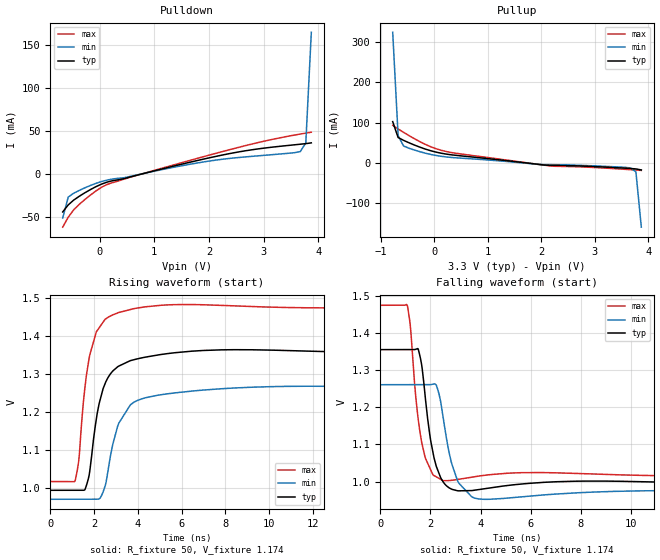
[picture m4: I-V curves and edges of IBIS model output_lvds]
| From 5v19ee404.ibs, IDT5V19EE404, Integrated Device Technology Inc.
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|   Model output_lvds
[Model]   output_lvds
Model_type   Output
Polarity   Non-Inverting
|   typ   min   max
C_comp   2pF   1.5pF   2.5pF
Vmeas = 1.13V
Rref = 50
Cref = 0
Vref = 1.13V
|   typ   min   max
[Voltage range]   3.3V   3.135V   3.465V
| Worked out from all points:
|   slope of the pulldown table from 0 to 0.495 V, typ, clamps not added: 59.8 ohm
|   slope of the pullup table from 0 to 0.495 V, typ, clamps not added: 47.6 ohm
|   rising waveform, R_fixture 50, V_fixture 1.174: 20-80 % time 714ps typ, 929ps min, 613ps max; typ from 0.993 V to 1.35 V
|   falling waveform, R_fixture 50, V_fixture 1.174: 20-80 % time 432ps typ, 501ps min, 405ps max; typ from 1.35 V to 0.993 V
[Pulldown]
|Voltage   I (typ)   I (min)   I (max)
|Note, modeling breaks down at 250mA and above.  This is well beyond the functional   |
|operating range of the device.  Should this scenario occur, catastrophic failure and   |
|possible damage to the device and/or board is of higher concern than the I-V curve   |
|behavior.  The IBIS checker will flag currents in excess of 10A with warnings.  Lines   |
|with currents in excess of 0.35 A have been commented out.  The points still remain|
|available to the user if the user desires to use them.   |
|-3.30000e+00   -6.87685e+01   -5.43171e+01   -9.32007e+01
|-3.19898e+00   -6.58202e+01   -5.20452e+01   -8.91014e+01
|-3.09796e+00   -6.28734e+01   -4.97746e+01   -8.50038e+01
|-2.99694e+00   -5.99283e+01   -4.75054e+01   -8.09081e+01
|-2.89592e+00   -5.69849e+01   -4.52379e+01   -7.68145e+01
|-2.79490e+00   -5.40436e+01   -4.29720e+01   -7.27232e+01
|-2.69388e+00   -5.11045e+01   -4.07081e+01   -6.86346e+01
|-2.59286e+00   -4.81679e+01   -3.84464e+01   -6.45488e+01
|-2.49184e+00   -4.52340e+01   -3.61870e+01   -6.04662e+01
|-2.39082e+00   -4.23033e+01   -3.39304e+01   -5.63874e+01
|-2.28980e+00   -3.93762e+01   -3.16768e+01   -5.23129e+01
|-2.18878e+00   -3.64533e+01   -2.94267e+01   -4.82434e+01
|-2.08776e+00   -3.35351e+01   -2.71806e+01   -4.41796e+01
|-1.98673e+00   -3.06226e+01   -2.49393e+01   -4.01228e+01
|-1.88571e+00   -2.77168e+01   -2.27034e+01   -3.60743e+01
|-1.78469e+00   -2.48193e+01   -2.04743e+01   -3.20362e+01
|-1.68367e+00   -2.19318e+01   -1.82533e+01   -2.80115e+01
|-1.58265e+00   -1.90572e+01   -1.60423e+01   -2.40041e+01
|-1.48163e+00   -1.61996e+01   -1.38443e+01   -2.00194e+01
|-1.38061e+00   -1.33650e+01   -1.16633e+01   -1.60669e+01
|-1.27959e+00   -1.05641e+01   -9.50588e+00   -1.21633e+01
|-1.17857e+00   -7.81468e+00   -7.38281e+00   -8.34234e+00
|-1.07755e+00   -5.15408e+00   -5.31429e+00   -4.68989e+00
|-9.76531e-01   -2.67976e+00   -3.34319e+00   -1.52157e+00
|-8.75510e-01   -7.34230e-01   -1.58050e+00   -1.40830e-01
|-7.74490e-01   -8.44745e-02   -3.68373e-01   -7.56037e-02
-673.5mV  -44.12mA   -51.13mA   -61.81mA
-572.4mV  -35.88mA   -26.81mA   -50.24mA
-471.4mV  -30.25mA   -22.24mA   -41.53mA
-370.4mV  -25.84mA   -19mA      -35.27mA
33.67mV   -11.77mA   -8.741mA   -15.46mA
538.8mV   -3.726mA   -3.071mA   -4.119mA
1.448V    10.68mA    9.012mA    12.28mA
2.256V    22.28mA    17.32mA    26.32mA
2.862V    28.96mA    21.02mA    36.12mA
3.67V     34.74mA    26.19mA    46.58mA
3.771V    35.43mA    36.18mA    47.67mA
3.872V    36.31mA    165mA      48.72mA
| 3.97347e+00   3.90604e-02   7.21592e-01   4.97824e-02
| 4.07449e+00   7.95512e-02   1.56794e+00   5.12016e-02
| 4.17551e+00   5.50354e-01   2.52334e+00   5.37009e-02
| 4.27653e+00   1.56933e+00   3.52849e+00   6.05171e-02
| 4.37755e+00   2.77655e+00   4.56116e+00   2.90811e-01
| 4.47857e+00   4.05579e+00   5.61110e+00   1.44560e+00
| 4.57959e+00   5.37132e+00   6.67281e+00   2.97907e+00
| 4.68061e+00   6.70844e+00   7.74304e+00   4.62016e+00
| 4.78163e+00   8.05979e+00   8.81972e+00   6.30839e+00
| 4.88265e+00   9.42118e+00   9.90143e+00   8.02268e+00
| 4.98367e+00   1.07900e+01   1.09873e+01   9.75343e+00
| 5.08469e+00   1.21646e+01   1.20769e+01   1.14955e+01
| 5.18571e+00   1.35438e+01   1.31697e+01   1.32457e+01
| 5.28673e+00   1.49267e+01   1.42651e+01   1.50023e+01
| 5.38776e+00   1.63127e+01   1.53626e+01   1.67637e+01
| 5.48878e+00   1.77013e+01   1.64619e+01   1.85291e+01
| 5.58980e+00   1.90921e+01   1.75627e+01   2.02978e+01
| 5.69082e+00   2.04848e+01   1.86650e+01   2.20692e+01
| 5.79184e+00   2.18792e+01   1.97684e+01   2.38429e+01
| 5.89286e+00   2.32754e+01   2.08729e+01   2.56187e+01
| 5.99388e+00   2.46734e+01   2.19784e+01   2.73961e+01
| 6.09490e+00   2.60729e+01   2.30848e+01   2.91751e+01
| 6.19592e+00   2.74736e+01   2.41920e+01   3.09553e+01
| 6.29694e+00   2.88754e+01   2.52999e+01   3.27368e+01
| 6.39796e+00   3.02780e+01   2.64085e+01   3.45193e+01
| 6.49898e+00   3.16814e+01   2.75177e+01   3.63028e+01
| 6.60000e+00   3.30855e+01   2.86274e+01   3.80871e+01
[Pullup]
|Voltage   I (typ)   I (min)   I (max)
|Note, modeling breaks down at 250mA and above.  This is well beyond the functional   |
|operating range of the device.  Should this scenario occur, catastrophic failure and   |
|possible damage to the device and/or board is of higher concern than the I-V curve   |
|behavior.  The IBIS checker will flag currents in excess of 10A with warnings.  Lines   |
|with currents in excess of 0.35 A have been commented out.  The points still remain|
|available to the user if the user desires to use them.   |
|-3.30000e+00   3.30649e+01   2.68016e+01   4.09786e+01
|-3.19898e+00   3.16617e+01   2.56933e+01   3.91941e+01
|-3.09796e+00   3.02592e+01   2.45857e+01   3.74103e+01
|-2.99694e+00   2.88577e+01   2.34787e+01   3.56274e+01
|-2.89592e+00   2.74574e+01   2.23726e+01   3.38453e+01
|-2.79490e+00   2.60586e+01   2.12672e+01   3.20642e+01
|-2.69388e+00   2.46610e+01   2.01628e+01   3.02842e+01
|-2.59286e+00   2.32645e+01   1.90595e+01   2.85054e+01
|-2.49184e+00   2.18693e+01   1.79573e+01   2.67280e+01
|-2.39082e+00   2.04756e+01   1.68564e+01   2.49522e+01
|-2.28980e+00   1.90836e+01   1.57571e+01   2.31782e+01
|-2.18878e+00   1.76934e+01   1.46596e+01   2.14063e+01
|-2.08776e+00   1.63054e+01   1.35644e+01   1.96368e+01
|-1.98673e+00   1.49200e+01   1.24719e+01   1.78702e+01
|-1.88571e+00   1.35377e+01   1.13822e+01   1.61071e+01
|-1.78469e+00   1.21590e+01   1.02955e+01   1.43482e+01
|-1.68367e+00   1.07850e+01   9.21254e+00   1.25947e+01
|-1.58265e+00   9.41664e+00   8.13421e+00   1.08481e+01
|-1.48163e+00   8.05582e+00   7.06175e+00   9.11072e+00
|-1.38061e+00   6.70508e+00   5.99695e+00   7.38625e+00
|-1.27959e+00   5.36863e+00   4.94257e+00   5.68119e+00
|-1.17857e+00   4.05393e+00   3.90315e+00   4.00831e+00
|-1.07755e+00   2.77593e+00   2.88682e+00   2.39814e+00
|-9.76531e-01   1.57108e+00   1.91017e+00   9.53385e-01
|-8.75510e-01   5.58820e-01   1.01408e+00   1.52918e-01
-774.5mV  102.2mA    323.4mA    93.03mA
-673.5mV  62.84mA    67.73mA    84.09mA
-572.4mV  55.86mA    41.9mA     75.76mA
-370.4mV  44.27mA    31.88mA    60.01mA
-67.35mV  30.17mA    20.96mA    40.14mA
134.7mV   23.86mA    16.26mA    31.05mA
336.7mV   19.73mA    13.3mA     25.29mA
2.155V    -6.05mA    -4.394mA   -7.483mA
2.963V    -8.992mA   -7.283mA   -11.27mA
3.67V     -13.9mA    -12.54mA   -16.81mA
3.771V    -15mA      -22.29mA   -17.68mA
3.872V    -17.52mA   -159.3mA   -18.74mA
| 3.97347e+00   -2.33400e-02   -1.03894e+00   -2.12284e-02
| 4.07449e+00   -6.44071e-02   -2.66328e+00   -2.74433e-02
| 4.17551e+00   -7.26444e-01   -4.57897e+00   -3.69091e-02
| 4.27653e+00   -2.67901e+00   -6.61921e+00   -5.08167e-02
| 4.37755e+00   -5.15548e+00   -8.72536e+00   -3.22188e-01
| 4.47857e+00   -7.81696e+00   -1.08716e+01   -2.57527e+00
| 4.57959e+00   -1.05668e+01   -1.30445e+01   -5.99938e+00
| 4.68061e+00   -1.33678e+01   -1.52365e+01   -9.73121e+00
| 4.78163e+00   -1.62020e+01   -1.74427e+01   -1.35885e+01
| 4.88265e+00   -1.90591e+01   -1.96600e+01   -1.75125e+01
| 4.98367e+00   -2.19330e+01   -2.18859e+01   -2.14777e+01
| 5.08469e+00   -2.48198e+01   -2.41190e+01   -2.54708e+01
| 5.18571e+00   -2.77167e+01   -2.63580e+01   -2.94842e+01
| 5.28673e+00   -3.06217e+01   -2.86020e+01   -3.35131e+01
| 5.38776e+00   -3.35335e+01   -3.08503e+01   -3.75539e+01
| 5.48878e+00   -3.64509e+01   -3.31022e+01   -4.16042e+01
| 5.58980e+00   -3.93731e+01   -3.53574e+01   -4.56623e+01
| 5.69082e+00   -4.22995e+01   -3.76153e+01   -4.97268e+01
| 5.79184e+00   -4.52294e+01   -3.98758e+01   -5.37968e+01
| 5.89286e+00   -4.81625e+01   -4.21385e+01   -5.78715e+01
| 5.99388e+00   -5.10984e+01   -4.44032e+01   -6.19502e+01
| 6.09490e+00   -5.40367e+01   -4.66697e+01   -6.60325e+01
| 6.19592e+00   -5.69773e+01   -4.89378e+01   -7.01179e+01
| 6.29694e+00   -5.99199e+01   -5.12074e+01   -7.42060e+01
| 6.39796e+00   -6.28643e+01   -5.34784e+01   -7.82967e+01
| 6.49898e+00   -6.58103e+01   -5.57507e+01   -8.23896e+01
| 6.60000e+00   -6.87579e+01   -5.80241e+01   -8.64845e+01
[Ramp]
|   typ   min   max
dV/dt_r   0.222/0.774n   0.178/0.949n   0.28/0.643n
dV/dt_f   0.229/0.48n   0.186/0.577n   0.284/0.436n
R_load =   50.0000
[Rising Waveform]
R_fixture = 50
V_fixture = 1.174   |Vcc_typ
V_fixture_min = 1.119 |Vcc_min
V_fixture_max = 1.245 |Vcc_max
C_fixture = 0.0p
| Time   typ   min   max
0s        992.9mV    969.2mV    1.016V
1.135ns   992.9mV    969.2mV    1.018V
1.313ns   992.9mV    969.2mV    1.077V
1.587ns   995.1mV    969.2mV    1.266V
1.807ns   1.044V     969.2mV    1.35V
2.235ns   1.222V     970.3mV    1.421V
2.762ns   1.301V     1.087V     1.452V
3.141ns   1.32V      1.171V     1.462V
4.353ns   1.344V     1.237V     1.476V
16ns      1.355V     1.265V     1.474V
[Falling Waveform]
R_fixture = 50
V_fixture = 1.174   |Vcc_typ
V_fixture_min = 1.119 |Vcc_min
V_fixture_max = 1.245 |Vcc_max
C_fixture = 0.0p
| Time   typ   min   max
0s        1.355V     1.261V     1.474V
1.082ns   1.355V     1.261V     1.473V
1.503ns   1.358V     1.261V     1.173V
1.773ns   1.241V     1.261V     1.07V
2.05ns    1.096V     1.261V     1.026V
2.235ns   1.041V     1.259V     1.013V
2.5ns     999.8mV    1.177V     1.003V
3.088ns   975.2mV    1.001V     1.006V
3.814ns   977.4mV    954.7mV    1.014V
16ns      992.6mV    973.1mV    1.016V
